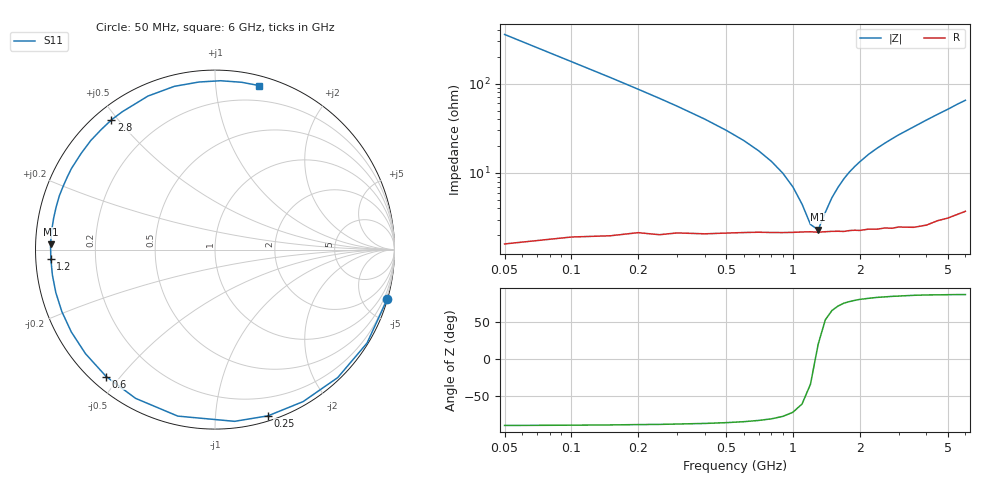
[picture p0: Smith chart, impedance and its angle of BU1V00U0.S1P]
! Infineon Technologies  Discrete & RF Semiconductors
! BB 833
! Si Tuning Diode in SOD323
! VR = 1 V
! S-Parameters:  June  1999
# GHz  S  MA  R  50
!  f  S11
! GHz  MAG  ANG
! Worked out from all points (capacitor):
!   34 points, 50 MHz to 6 GHz, reference 50 ohm
!   read as one part to ground: C = 8.93 pF near 50 MHz
!   lowest |Z| = 2.31 ohm at 1.3 GHz (marker M1)
!   series resonance near 1.265 GHz, so ESL is about 1.8 nH
!   S11 on the Smith chart (normalised r, x): 50 MHz: 0.03, -7.12; 250 MHz: 0.04, -1.37; 600 MHz: 0.04, -0.46; 1.2 GHz: 0.04, -0.03; 2.8 GHz: 0.05, +0.48; 6 GHz: 0.07, +1.30
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0.05  0.9988 -16.0
0.1  0.9943 -31.6
0.15  0.9879 -46.2
0.2  0.9789 -59.9
0.25  0.9721 -72.3
0.3  0.963 -83.5
0.4  0.9506 -102.6
0.5  0.9395 -118.1
0.6  0.9315 -130.6
0.7  0.9258 -141.2
0.8  0.9228 -150.2
0.9  0.9205 -158.0
1  0.9186 -164.9
1.2  0.9161 -176.6
1.3  0.9169 178.2
1.4  0.9162 173.4
1.6  0.9163 165.0
1.8  0.9167 157.3
2  0.9186 150.6
2.4  0.9211 138.7
2.8  0.925 128.6
3  0.9256 123.9
3.5  0.9334 113.6
4  0.9374 104.0
4.5  0.938 95.5
5  0.9414 88.1
5.5  0.944 80.9
6  0.9464 75.0
